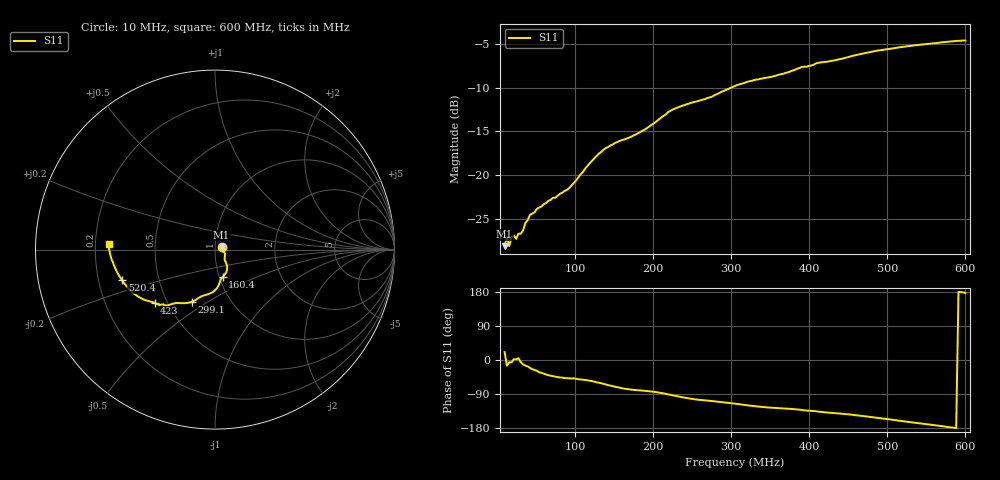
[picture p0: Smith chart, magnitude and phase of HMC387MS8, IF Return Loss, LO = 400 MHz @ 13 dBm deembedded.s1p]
!Hittite Microwave Corporation
!12 Elizabeth Drive
!Chelmsford, MA 01824
!Tel: 978-250-3343
!Fax: 978-250-3373
!Device: HMC387MS8, 450-500 MHz, GaAs MMIC High IP3 Mixer in 8-lead plastic SMT package
!Misc: IF Return Loss, LO = 400 MHz @ 13 dBm, Room
# MHZ S MA R 50
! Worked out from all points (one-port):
!   201 points, 10 MHz to 600 MHz, reference 50 ohm
!   lowest |S11| = -28.2 dB at 10 MHz (marker M1), VSWR 1.08, Z = 53.8 + j1.5 ohm
!   |S11| at or under -10 dB: start of sweep to 299.2 MHz
!   S11 on the Smith chart (normalised r, x): 10 MHz: 1.08, +0.03; 160.4 MHz: 1.04, -0.33; 299.1 MHz: 0.66, -0.43; 423 MHz: 0.43, -0.32; 520.4 MHz: 0.30, -0.15; 600 MHz: 0.26, +0.02
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10  0.039 20.9
12.95  0.044 -14.9
15.9  0.039 -5.9
18.85  0.044 -6.3
21.8  0.045 2.2
24.75  0.043 1.7
27.7  0.046 4.8
30.65  0.046 -5.6
42.45  0.059 -21.0
83.75  0.079 -46.4
92.6  0.084 -48.3
130.95  0.133 -60.1
157.5  0.157 -73.2
160.45  0.159 -74.7
178.15  0.171 -79.3
201.75  0.199 -84.0
231.25  0.244 -95.8
275.5  0.282 -108.4
299.1  0.316 -113.7
305  0.325 -115.2
378.75  0.398 -129.4
423  0.448 -138.7
452.5  0.479 -143.9
484.95  0.516 -152.0
520.35  0.545 -161.7
526.25  0.55 -163.2
573.45  0.581 -175.8
600  0.592 177.0
